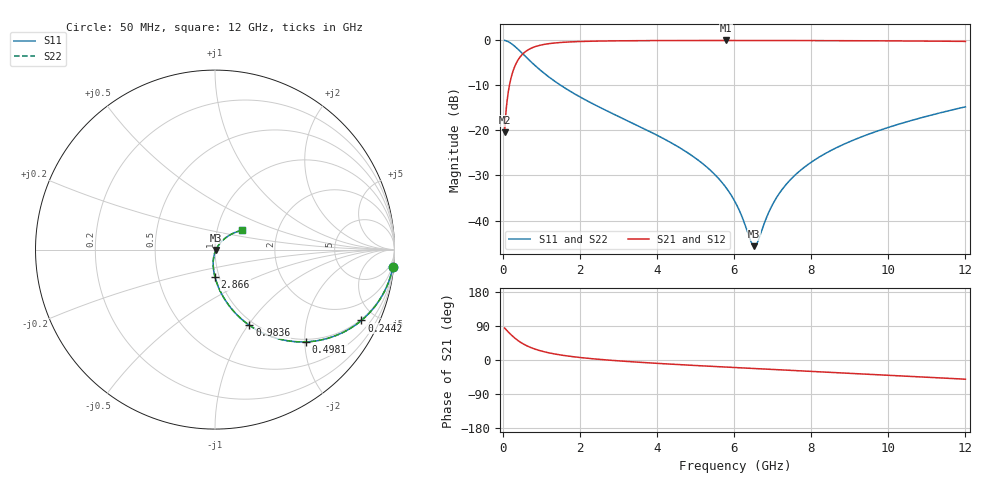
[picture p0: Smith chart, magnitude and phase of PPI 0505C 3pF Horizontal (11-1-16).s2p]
# MHz S MA R 50
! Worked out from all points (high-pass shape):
!   1601 points, 50 MHz to 12 GHz, reference 50 ohm
!   highest |S21| = -0.05 dB at 5.801 GHz (marker M1); lowest = -20.5 dB at 50 MHz (marker M2)
!   |S21| within 3 dB of the highest: 519.4 MHz to end of sweep
!   lowest |S11| = -45.7 dB at 6.525 GHz (marker M3), VSWR 1.01, Z = 50.5 - j0.216 ohm
!   |S11| at or under -10 dB: 1.507 GHz to end of sweep
!   |S22| runs from -45.7 to 0.0 dB; largest |S21 - S12| = 0
!   S11 on the Smith chart (normalised r, x): 50 MHz: 1, -20; 244.2 MHz: 0.94, -4.16; 498.1 MHz: 0.94, -2.03; 983.6 MHz: 0.94, -1.02; 2.866 GHz: 0.95, -0.30; 12 GHz: 1.31, +0.29
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50  0.9955 -5.6  0.09484 84.4  0.09484 84.4  0.9955 -5.6
154.5625  0.9591 -17.0  0.2826 73.0  0.2826 73.0  0.9591 -17.0
244.1875  0.9061 -25.8  0.422 64.1  0.422 64.1  0.9061 -25.8
498.125  0.723 -45.3  0.6891 44.6  0.6891 44.6  0.723 -45.3
722.1875  0.5834 -56.6  0.81 33.2  0.81 33.2  0.5834 -56.6
983.5938  0.4636 -65.5  0.8836 24.2  0.8836 24.2  0.4636 -65.5
1416.781  0.3356 -74.9  0.9393 14.7  0.9393 14.7  0.3356 -74.9
2044.156  0.2302 -83.1  0.9701 6.2  0.9701 6.2  0.2302 -83.1
2865.719  0.1524 -90.0  0.985 -1.2  0.985 -1.2  0.1524 -90.0
4038.312  0.08686 -96.6  0.9923 -9.1  0.9923 -9.1  0.08686 -96.6
5106.344  0.04553 -99.7  0.9944 -15.1  0.9944 -15.1  0.04553 -99.7
5800.938  0.02293 -96.9  0.9947 -18.8  0.9947 -18.8  0.02293 -96.9
6025  0.01617 -92.5  0.9947 -19.9  0.9947 -19.9  0.01617 -92.5
6435.781  0.005873 -51.3  0.9945 -22.0  0.9945 -22.0  0.005873 -51.3
6525.406  0.005191 -24.3  0.9944 -22.5  0.9944 -22.5  0.005191 -24.3
6607.562  0.00573 0.8  0.9943 -22.9  0.9943 -22.9  0.00573 0.8
6906.312  0.01249 39.6  0.994 -24.4  0.994 -24.4  0.01249 39.6
7175.188  0.02004 47.8  0.9937 -25.8  0.9937 -25.8  0.02004 47.8
8019.156  0.04486 51.9  0.9921 -30.0  0.9921 -30.0  0.04486 51.9
8870.594  0.07094 49.9  0.9898 -34.3  0.9898 -34.3  0.07094 49.9
10013.31  0.1083 45.5  0.9852 -40.1  0.9852 -40.1  0.1083 45.5
12000  0.1826 35.9  0.9717 -50.7  0.9717 -50.7  0.1826 35.9
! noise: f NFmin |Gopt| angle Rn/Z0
50  0.0009765  0.9483  1.1  0.004238
1372  0.006189  0.7777  5.471  0.005685
2701  0.00927  0.7181  9.954  0.006457
4031  0.01228  0.6893  14.36  0.007572
5360  0.01546  0.6766  18.72  0.008993
6682  0.01884  0.6728  22.99  0.01066
8012  0.02249  0.6745  27.22  0.01261
9341  0.02643  0.68  31.38  0.01485
1.067e+04  0.03071  0.6882  35.47  0.01743
1.2e+04  0.03539  0.6985  39.47  0.02042
